(* Logix 5000 AddOnInstructionDefinition export NORD_ADC; software revision 24.02 *)

TYPE NORD_ParameterBackup :
STRUCT
   DeviceID : STRING;   // Device ID of VFD
   MacAddress : SINT[6];   // MAC Address of CU/TU
   ParamVFD : NORD_ParameterStoreInfo[1650];   // VFD Parameter Backup Values
   ParamCTU : NORD_ParameterStoreInfo[150];   // CU4/TU4 Parameter Backup Values
   HasIntPLC : BOOL;   // VFD contains an internal PLC Program
END_STRUCT
END_TYPE

TYPE NORD_ParameterStoreInfo :
STRUCT
   Num : INT;
   Inst : INT;
   Value : DINT;
END_STRUCT
END_TYPE

ADD_ON_INSTRUCTION NORD_ADC   (* revision 1.0, vendor NORD Drivesystems, ExecutePrescan, ExecuteEnableInFalse *)
// NORD ADC & Acyclic Comms.
// Revision note:
// For use with all NORD VFDs
//    - NORD Automatic Device Configurator
//       - Backup/Restore Parameters
//    - Acyclic Comms. for Parameter Read/Write
// Created By: Adam Desouky
VAR_IN_OUT
   ModuleName : MODULE; {required}
END_VAR
VAR_INPUT
   VFD_Number : SINT := 1; {visible}   // VFD Number in Localbus
   ParameterNumber : INT; {visible}
   ParameterIndex : SINT; {visible}
   ParameterSet : SINT; {visible}
END_VAR
VAR_OUTPUT
   Done : BOOL; {access Read Only, visible}
   Busy : BOOL; {access Read Only, visible}
END_VAR
VAR_IN_OUT
   ReadMsg : MESSAGE; {required}   // Read Msg to Module
END_VAR
VAR_INPUT
   ReadTrigger : BOOL; {visible}
   ReadValue : DINT; {access None, visible}   // Read Value from message
END_VAR
VAR_IN_OUT
   WriteMsg : MESSAGE; {required}   // Write Msg to Module
END_VAR
VAR_INPUT
   WriteTrigger : BOOL; {visible}
   WriteValue : DINT; {visible}
END_VAR
VAR_OUTPUT
   Error : BOOL; {access Read Only, visible}
   VFD_NotPresent : BOOL; {access Read Only, visible}   // VFD not present in Localbus
   EthernetDisconnected : BOOL; {access Read Only, visible}   // Eth. cord to Module is disconnected
END_VAR
VAR_IN_OUT
   Backup : NORD_ParameterBackup; {required}   // Parameter Backup File
END_VAR
VAR_OUTPUT
   CompletionPercent : DINT; {access None, visible}   // Backup/Restore Complete Percentage
   FirmwareUpdateRequired : BOOL; {access Read Only, visible}   // Parameter 780 not present
   NewDriveDetected : BOOL; {access Read Only, visible}   // New Device ID detected
   NewCTUnitDetected : BOOL; {access Read Only, visible}
END_VAR
VAR_INPUT
   BackupTrigger : BOOL; {visible}   // Trigger to start backing up the VFD parameters
   RestoreTrigger : BOOL; {visible}   // Trigger to start restoring the VFD parameters
   AutomaticRestore : BOOL; {access None, visible}   // Restore Automatically when New Drive is Detected
END_VAR
VAR_OUTPUT
   GetID_InProcess : BOOL; {access None, visible}
   BackupInProcess : BOOL; {access None, visible}
   RestoreInProcess : BOOL; {access None, visible}
   HasInternalPLC : BOOL; {access None, visible}
   ErrorID : DINT; {access Read Only, visible}   // Message Error Code
END_VAR
VAR_INPUT
   WriteValueMSG : DINT;
   ReadValueCarryOver : DINT; {access None}   // Do Not Delete
END_VAR
VAR
   ModulePath : SINT[32]; {access None}
   IP_Address : STRING; {access None}
   IP_Length : INT; {access None}
   Instance : INT;
   VFD_NumPrev : SINT := 1; {access None}
   VFD_NumLock : SINT := 1; {access None}
   GetID_SM : INT; {access None}   // 0: Not Active 10: Reset Info 20: Prepare Read Msg 30: Read Trigger 40: Read Complete 41: Store Data 42: Record Error 50: Increment Index 51: Switch to CU/TU
   HasParamIndex : BOOL; {access None}   // Set Parameter has Indexes
   HasParamSets : BOOL; {access None}   // Set Parameter has Parameter Sets
   ReadErrorOS : BOOL; {access None}
   WriteErrorONS : BOOL; {access None}
   TrigONS1 : BOOL; {access None}
   ReadDoneOS : BOOL; {access None}
   WriteDoneONS : BOOL; {access None}
   FaultCode : DINT; {access None}
   MacAddr : SINT[6]; {access None}   // MAC Address of CU/TU
   GetID_ReadTrigger : BOOL; {access None}
   EthConnONS : BOOL; {access None}
   GetID_DoneONS : BOOL; {access None}
   BackupSM : INT; {access None}   // 0: Not Active 10: Reset indexes 20: Clear Old Backup 30: Reset Indexes 40: Prepare Read Msg 50: Read Trigger 60: Read Complete 61: Store Data 70/71: Increment Store index/Instance 80: Increment Param 90: Store Device ID
   Index : INT; {access None}
   DeviceID : STRING; {access None}   // Device ID of VFD
   RestoreSM : INT; {access None}   // 0: Not Active 10: Reset Indexes 15: # of Saved Param 20: Get RestoreParam 21: Prepare Read Msg 22: Read Trigger 23: Read Complete 24: Compare Data 30: Prepare WriteMsg 40: Write Trigger 50: Write Complete 60: Inc. Store Index 70: Store Devide ID
   Index1 : INT; {access None}   // Store Index: VFD
   IndexInst : INT; {access None}   // Instance Index
   RestoreParam : INT := 5; {access None}   // Parameter Number to be Restored
   SavedParamsVFD : INT; {access None}
   MaxIndexVFD : INT; {access None}   // Maximun possible stored parameters
   BackupReadTrigger : BOOL; {access None}
   BackupIndexONS : BOOL; {access None}
   StartBackupONS : BOOL; {access None}
   RestWriteTrig : BOOL; {access None}
   RestIndexONS : BOOL; {access None}
   RestReadTrig : BOOL; {access None}
   BackupLast : BOOL; {access None}   // Determines Backup/Restore Complete Percentage Calculation
   WriteSM : SINT; {access None}   // 0: Not Active 10: Write LEN=4 20: 1st WriteTrigger 30: Write Complete - 40: Write LEN=2 - 50: 2nd WriteTrigger 60: Write Complete
   ID_Length : SINT := 12; {access None}
   Class : INT; {access None}
   TrigONS2 : BOOL; {access None}
   NullString : STRING; {access None}
   NumOfParams : DINT; {access None}   // Number of parameters in the VFD
   NewVFD_NumONS : BOOL; {access None}
   WriteTriggerONS : BOOL; {access None}
   WriteTrigInternal : BOOL; {access None}   // 1st Attempt: LEN = 4 2nd Attempt: LEN = 2
   Write16Bit : BOOL; {access None}   // 0: Write LEN=4 1: Write LEN=2
   AOI_FirstScan : BOOL; {access None}   // First Scan of AOI
   AOI_FirstScanONS : BOOL; {access None}
   Percent100ONS : BOOL; {access None}
   GetID_Done_ONS : BOOL; {access None}
   GetCTU_ID : BOOL; {access None}
   MaxIndexCTU : INT; {access None}
   Index2 : INT; {access None}   // Store Index: CU/TU
   SavedParamsCTU : INT; {access None}
   ID_Class : INT; {access None}
   RestoreCTU : BOOL; {access None}   // Restore CTU Parameters
   RestIndexONS2 : BOOL; {access None}
   ID_Attribute : INT; {access None}
   CompPercentIndex : INT; {access None}
   FirmwareONS : BOOL; {access None}
   StoreDevID : BOOL; {access None}
   StoreDevID_DN : BOOL; {access None}
   ResetIndexes : BOOL; {access None}
   ResetIndexDN : BOOL; {access None}
   GetRestParam : BOOL; {access None}   // Get Restore Parameter Logic
   GetRestParamDN : BOOL; {access None}   // Got Restore Param
   ClearDevID : BOOL; {access None}
   ClearDevID_DN : BOOL; {access None}
   ResetMsgEr : BOOL; {access None}
   ModuleEIP : BOOL; {access None}
   PerformRestoreONS : BOOL; {access None}
   RestoreFailed : BOOL; {access None}   // All writes in restore failed
   RestoreFailedONS : BOOL; {access None}
   RestoreHasWrite : BOOL; {access None}
   RestoreHasWriteONS : BOOL; {access None}
   AutomaticRestoreONS : BOOL; {access None}
   ModuleEIP_ONS : BOOL; {access None}
   GetID_Done : BOOL; {access None}
END_VAR

ROUTINE EnableInFalse   (* ladder *)
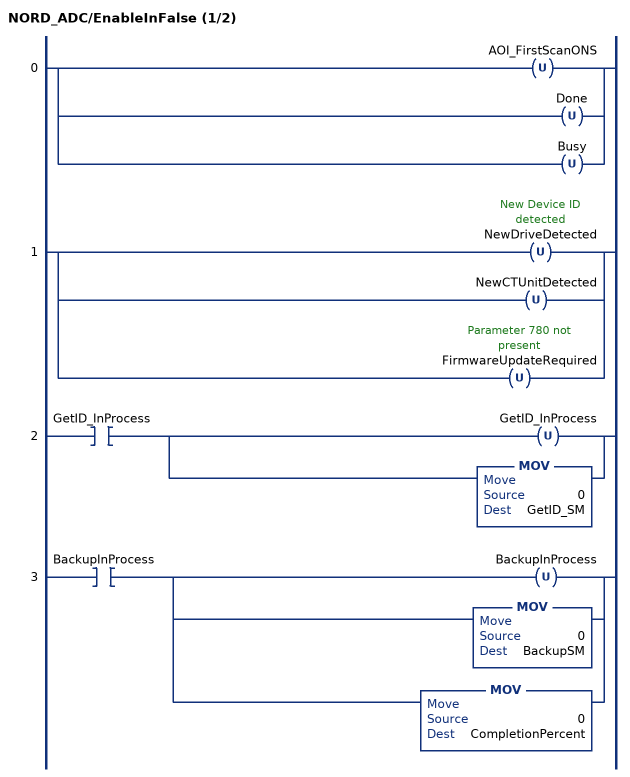
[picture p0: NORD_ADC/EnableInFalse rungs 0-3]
   0: [OTU(AOI_FirstScanONS) ,OTU(Done) ,OTU(Busy) ];
   1: [OTU(NewDriveDetected) ,OTU(NewCTUnitDetected) ,OTU(FirmwareUpdateRequired) ];
   2: XIC(GetID_InProcess)[OTU(GetID_InProcess) ,MOV(0,GetID_SM) ];
   3: XIC(BackupInProcess)[OTU(BackupInProcess) ,MOV(0,BackupSM) ,MOV(0,CompletionPercent) ];
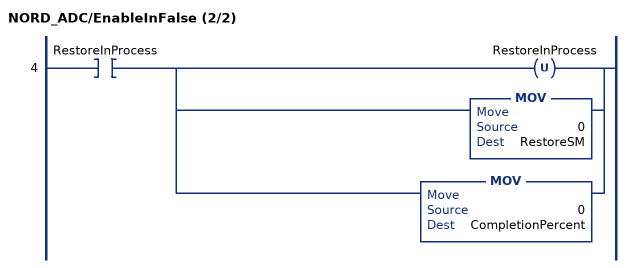
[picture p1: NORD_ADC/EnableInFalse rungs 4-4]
   4: XIC(RestoreInProcess)[OTU(RestoreInProcess) ,MOV(0,RestoreSM) ,MOV(0,CompletionPercent) ];
END_ROUTINE

ROUTINE Logic   (* ladder *)
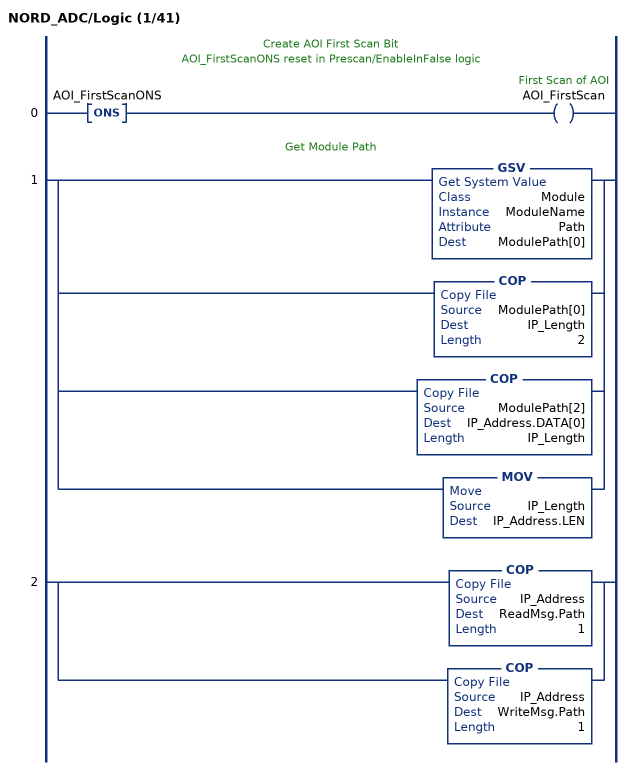
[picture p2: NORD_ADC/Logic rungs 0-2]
   // Create AOI First Scan Bit
   // AOI_FirstScanONS reset in Prescan/EnableInFalse logic
   0: ONS(AOI_FirstScanONS)OTE(AOI_FirstScan);
   // Get Module Path
   1: [GSV(Module,ModuleName,Path,ModulePath[0]) ,COP(ModulePath[0],IP_Length,2) ,COP(ModulePath[2],IP_Address.DATA[0],IP_Length) ,MOV(IP_Length,IP_Address.LEN) ];
   2: [COP(IP_Address,ReadMsg.Path,1) ,COP(IP_Address,WriteMsg.Path,1) ];
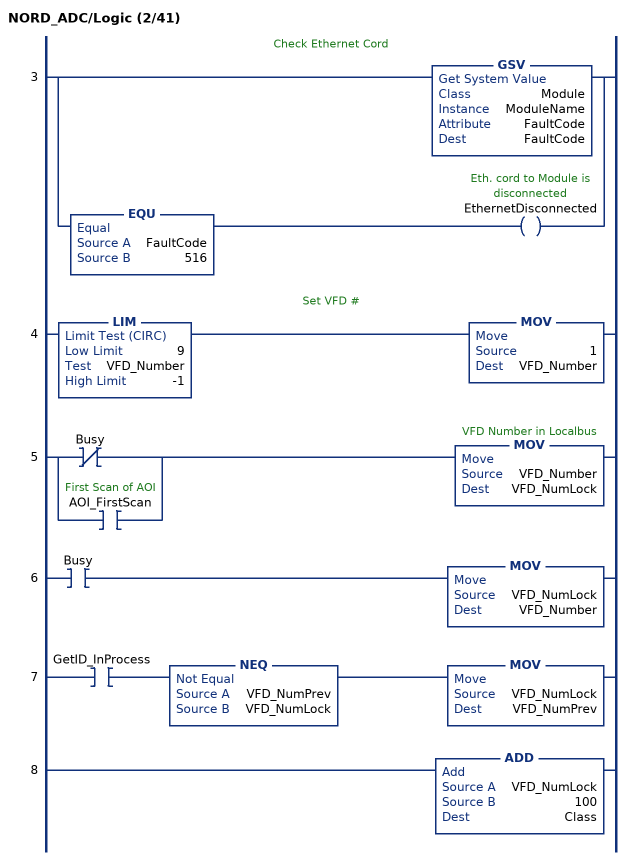
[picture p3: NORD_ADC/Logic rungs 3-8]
   // Check Ethernet Cord
   3: [GSV(Module,ModuleName,FaultCode,FaultCode) ,EQU(FaultCode,516) OTE(EthernetDisconnected) ];
   // Set VFD #
   4: LIM(9,VFD_Number,-1)MOV(1,VFD_Number);
   5: [XIO(Busy) ,XIC(AOI_FirstScan) ]MOV(VFD_Number,VFD_NumLock);
   6: XIC(Busy)MOV(VFD_NumLock,VFD_Number);
   7: XIC(GetID_InProcess)NEQ(VFD_NumPrev,VFD_NumLock)MOV(VFD_NumLock,VFD_NumPrev);
   8: ADD(VFD_NumLock,100,Class);
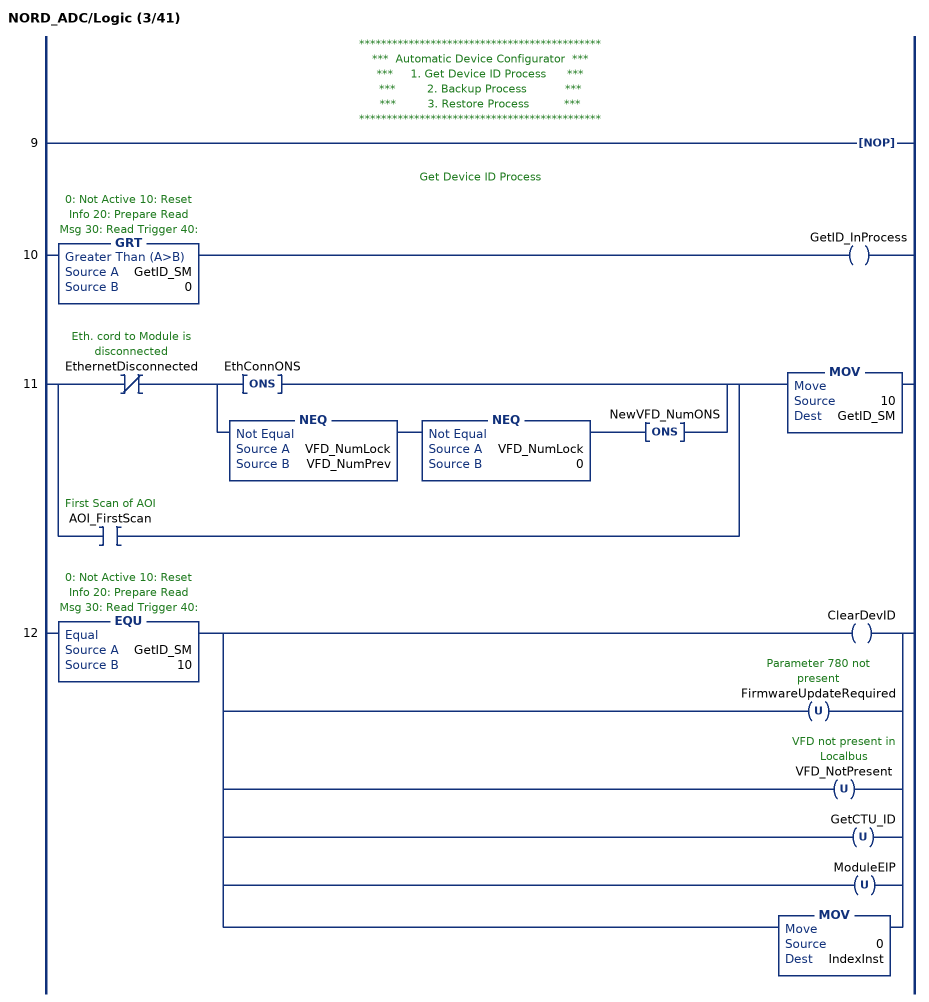
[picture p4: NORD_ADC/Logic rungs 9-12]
   // ********************************************
   // ***  Automatic Device Configurator  ***
   // ***     1. Get Device ID Process      ***
   // ***         2. Backup Process           ***
   // ***         3. Restore Process          ***
   // ********************************************
   9: NOP();
   // Get Device ID Process
   10: GRT(GetID_SM,0)OTE(GetID_InProcess);
   11: [XIO(EthernetDisconnected) [ONS(EthConnONS) ,NEQ(VFD_NumLock,VFD_NumPrev) NEQ(VFD_NumLock,0) ONS(NewVFD_NumONS) ] ,XIC(AOI_FirstScan) ]MOV(10,GetID_SM);
   12: EQU(GetID_SM,10)[OTE(ClearDevID) ,[OTU(FirmwareUpdateRequired) ,OTU(VFD_NotPresent) ,OTU(GetCTU_ID) ,OTU(ModuleEIP) ] ,MOV(0,IndexInst) ];
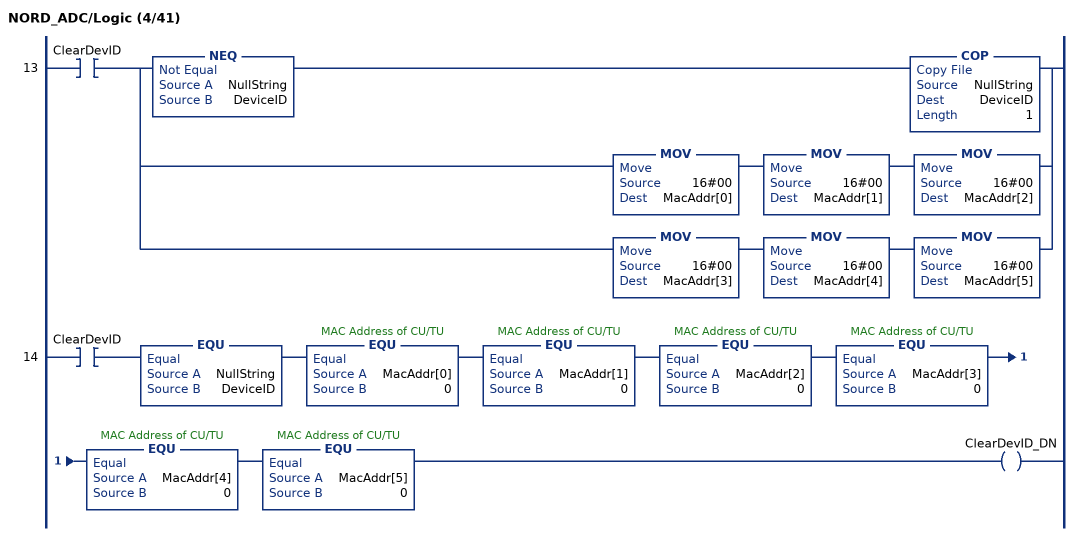
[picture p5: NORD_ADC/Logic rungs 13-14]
   13: XIC(ClearDevID)[NEQ(NullString,DeviceID) COP(NullString,DeviceID,1) ,MOV(16#00,MacAddr[0]) MOV(16#00,MacAddr[1]) MOV(16#00,MacAddr[2]) ,MOV(16#00,MacAddr[3]) MOV(16#00,MacAddr[4]) MOV(16#00,MacAddr[5]) ];
   14: XIC(ClearDevID)EQU(NullString,DeviceID)EQU(MacAddr[0],0)EQU(MacAddr[1],0)EQU(MacAddr[2],0)EQU(MacAddr[3],0)EQU(MacAddr[4],0)EQU(MacAddr[5],0)OTE(ClearDevID_DN);
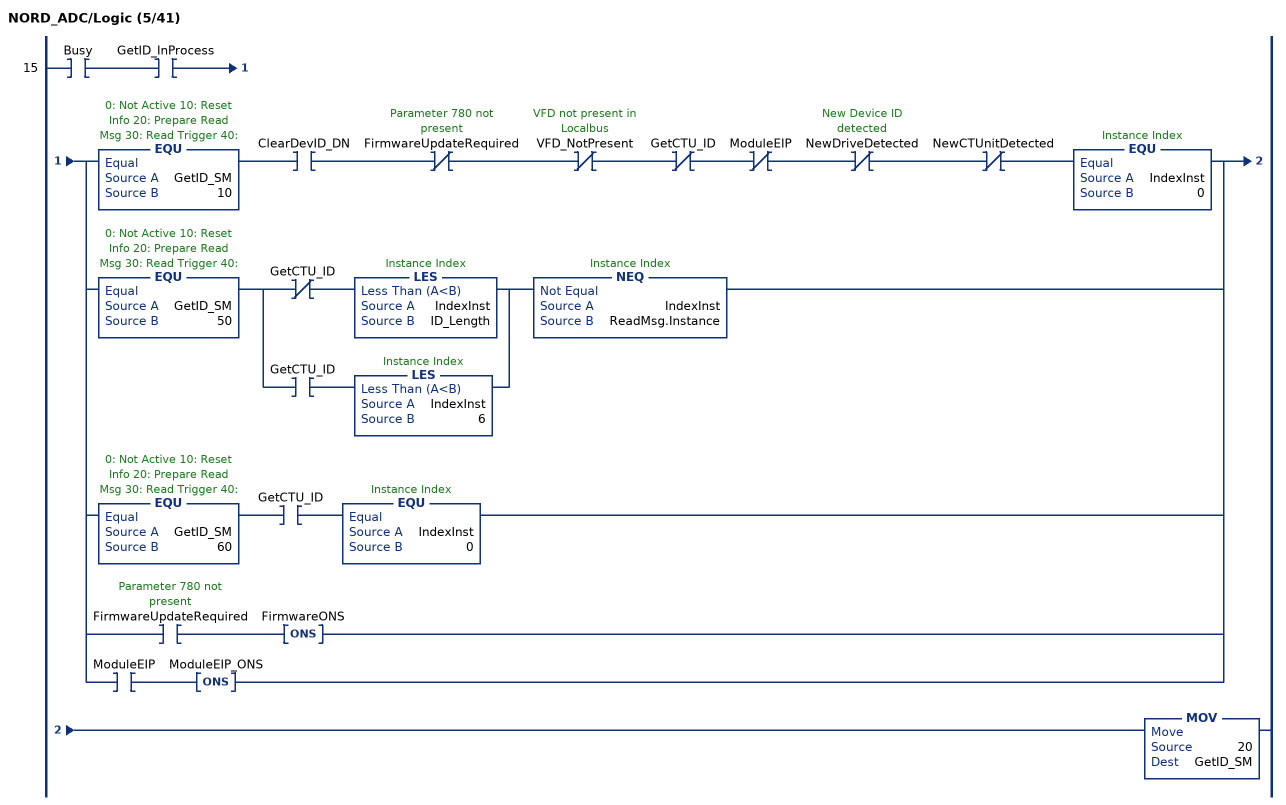
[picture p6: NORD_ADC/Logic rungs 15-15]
   15: XIC(Busy)XIC(GetID_InProcess)[EQU(GetID_SM,10) XIC(ClearDevID_DN) XIO(FirmwareUpdateRequired) XIO(VFD_NotPresent) XIO(GetCTU_ID) XIO(ModuleEIP) XIO(NewDriveDetected) XIO(NewCTUnitDetected) EQU(IndexInst,0) ,EQU(GetID_SM,50) [XIO(GetCTU_ID) LES(IndexInst,ID_Length) ,XIC(GetCTU_ID) LES(IndexInst,6) ] NEQ(IndexInst,ReadMsg.Instance) ,EQU(GetID_SM,60) XIC(GetCTU_ID) EQU(IndexInst,0) ,XIC(FirmwareUpdateRequired) ONS(FirmwareONS) ,XIC(ModuleEIP) ONS(ModuleEIP_ONS) ]MOV(20,GetID_SM);
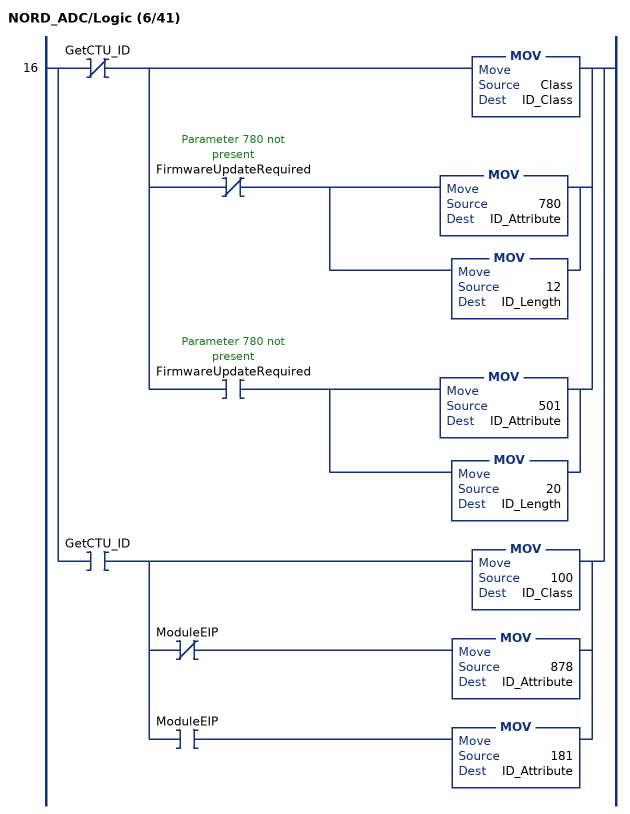
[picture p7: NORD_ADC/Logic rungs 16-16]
   16: [XIO(GetCTU_ID) [MOV(Class,ID_Class) ,XIO(FirmwareUpdateRequired) [MOV(780,ID_Attribute) ,MOV(12,ID_Length) ] ,XIC(FirmwareUpdateRequired) [MOV(501,ID_Attribute) ,MOV(20,ID_Length) ] ] ,XIC(GetCTU_ID) [MOV(100,ID_Class) ,XIO(ModuleEIP) MOV(878,ID_Attribute) ,XIC(ModuleEIP) MOV(181,ID_Attribute) ] ];
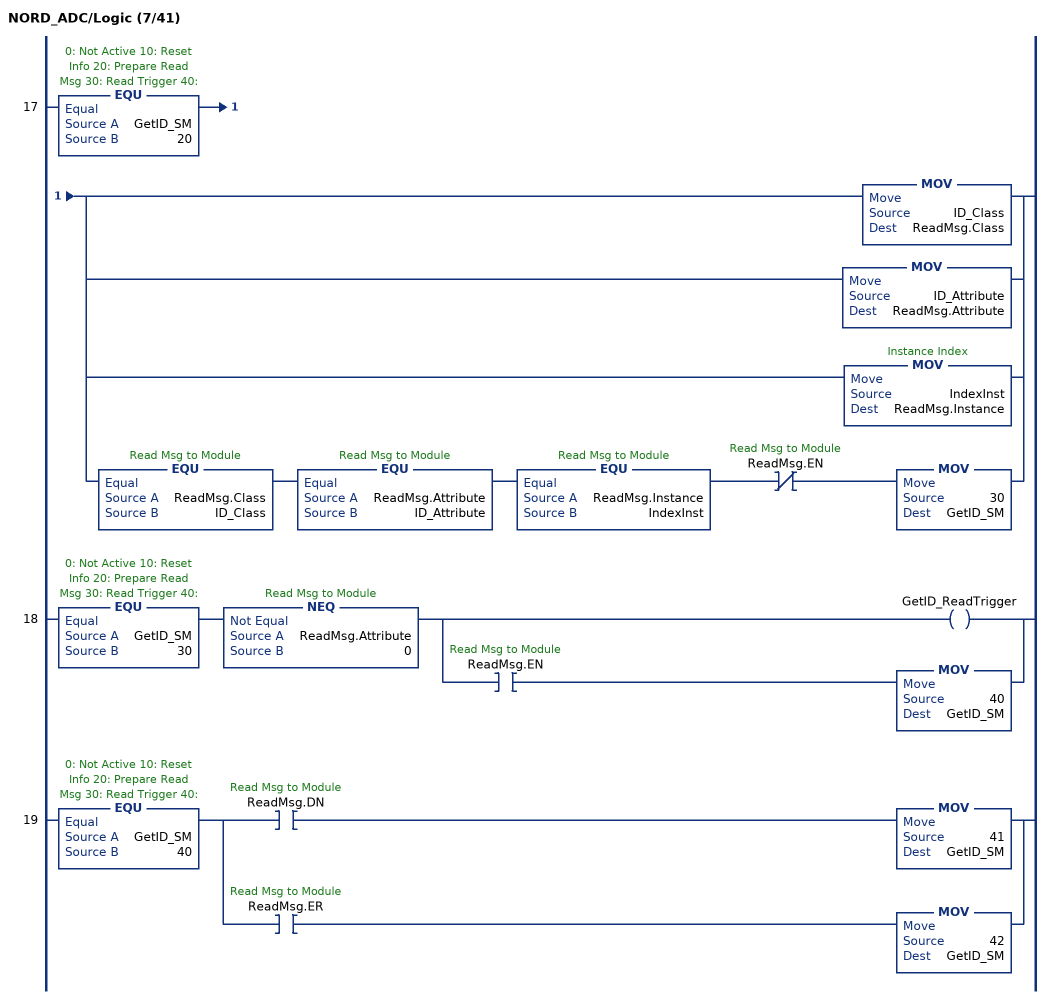
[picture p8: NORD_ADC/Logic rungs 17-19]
   17: EQU(GetID_SM,20)[[MOV(ID_Class,ReadMsg.Class) ,MOV(ID_Attribute,ReadMsg.Attribute) ,MOV(IndexInst,ReadMsg.Instance) ] ,EQU(ReadMsg.Class,ID_Class) EQU(ReadMsg.Attribute,ID_Attribute) EQU(ReadMsg.Instance,IndexInst) XIO(ReadMsg.EN) MOV(30,GetID_SM) ];
   18: EQU(GetID_SM,30)NEQ(ReadMsg.Attribute,0)[OTE(GetID_ReadTrigger) ,XIC(ReadMsg.EN) MOV(40,GetID_SM) ];
   19: EQU(GetID_SM,40)[XIC(ReadMsg.DN) MOV(41,GetID_SM) ,XIC(ReadMsg.ER) MOV(42,GetID_SM) ];
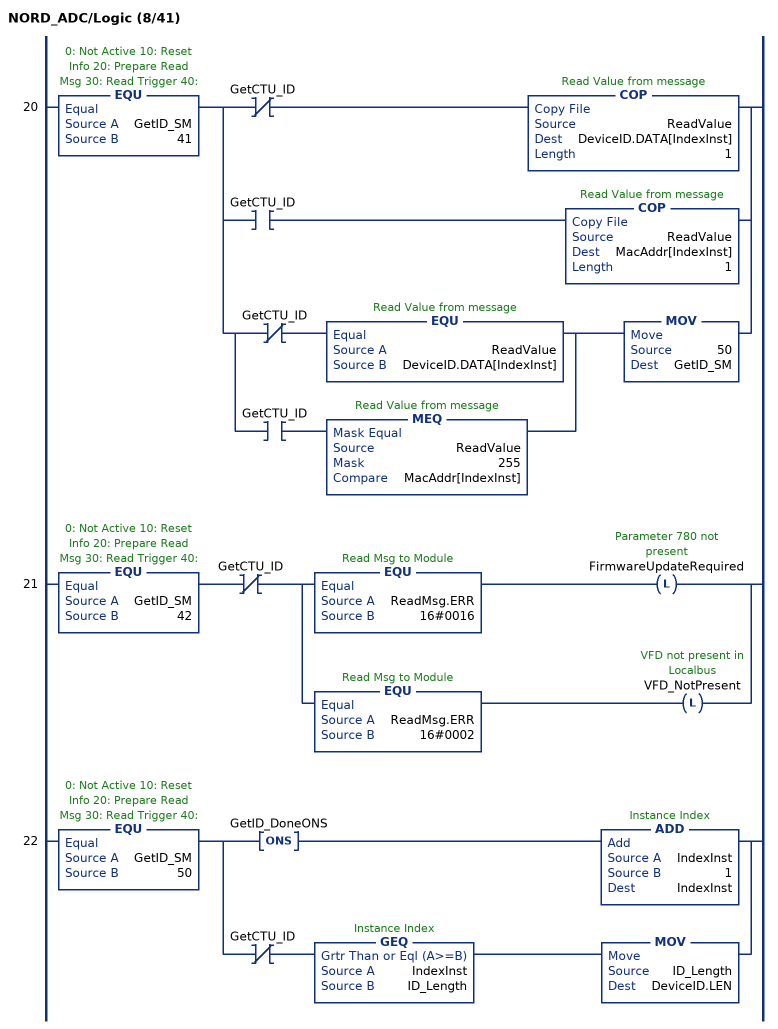
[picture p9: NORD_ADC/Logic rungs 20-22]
   20: EQU(GetID_SM,41)[[XIO(GetCTU_ID) COP(ReadValue,DeviceID.DATA[IndexInst],1) ,XIC(GetCTU_ID) COP(ReadValue,MacAddr[IndexInst],1) ] ,[XIO(GetCTU_ID) EQU(ReadValue,DeviceID.DATA[IndexInst]) ,XIC(GetCTU_ID) MEQ(ReadValue,255,MacAddr[IndexInst]) ] MOV(50,GetID_SM) ];
   21: EQU(GetID_SM,42)XIO(GetCTU_ID)[EQU(ReadMsg.ERR,16#0016) OTL(FirmwareUpdateRequired) ,EQU(ReadMsg.ERR,16#0002) OTL(VFD_NotPresent) ];
   22: EQU(GetID_SM,50)[ONS(GetID_DoneONS) ADD(IndexInst,1,IndexInst) ,XIO(GetCTU_ID) GEQ(IndexInst,ID_Length) MOV(ID_Length,DeviceID.LEN) ];
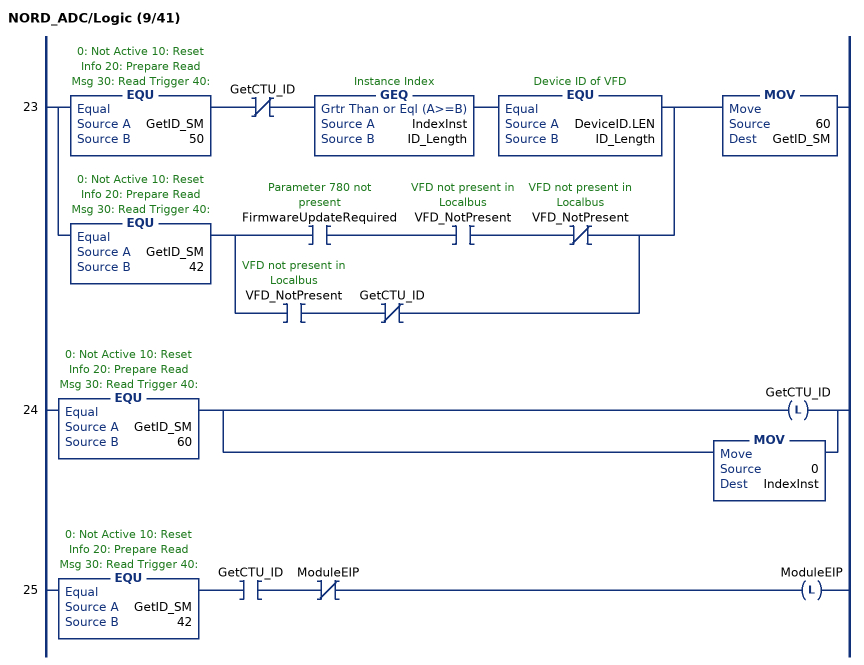
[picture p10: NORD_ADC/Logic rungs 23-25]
   23: [EQU(GetID_SM,50) XIO(GetCTU_ID) GEQ(IndexInst,ID_Length) EQU(DeviceID.LEN,ID_Length) ,EQU(GetID_SM,42) [XIC(FirmwareUpdateRequired) XIC(VFD_NotPresent) XIO(VFD_NotPresent) ,XIC(VFD_NotPresent) XIO(GetCTU_ID) ] ]MOV(60,GetID_SM);
   24: EQU(GetID_SM,60)[OTL(GetCTU_ID) ,MOV(0,IndexInst) ];
   25: EQU(GetID_SM,42)XIC(GetCTU_ID)XIO(ModuleEIP)OTL(ModuleEIP);
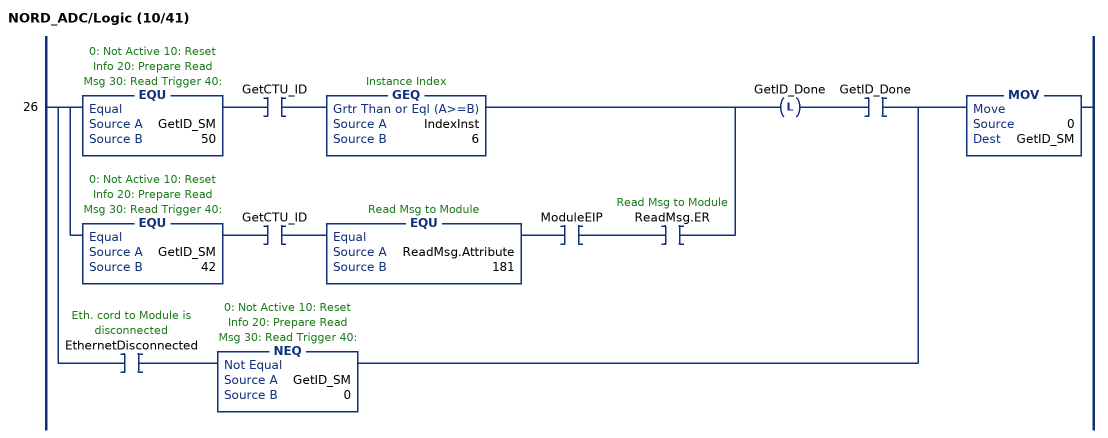
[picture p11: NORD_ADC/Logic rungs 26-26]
   26: [[EQU(GetID_SM,50) XIC(GetCTU_ID) GEQ(IndexInst,6) ,EQU(GetID_SM,42) XIC(GetCTU_ID) EQU(ReadMsg.Attribute,181) XIC(ModuleEIP) XIC(ReadMsg.ER) ] OTL(GetID_Done) XIC(GetID_Done) ,XIC(EthernetDisconnected) NEQ(GetID_SM,0) ]MOV(0,GetID_SM);
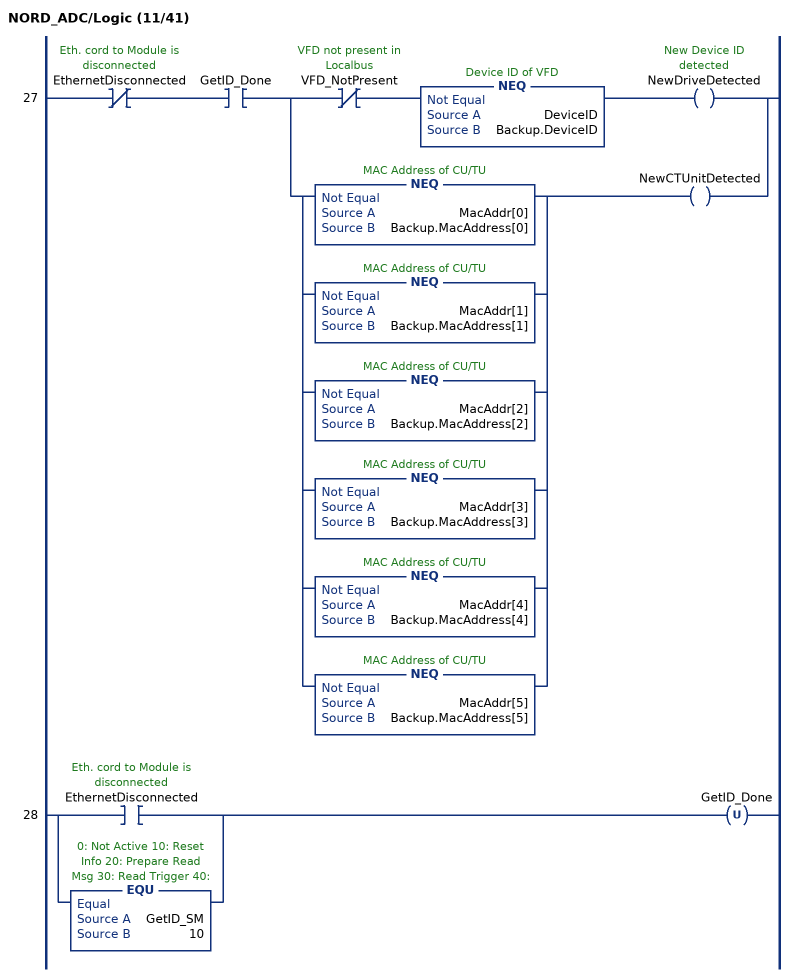
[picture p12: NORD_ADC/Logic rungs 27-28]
   27: XIO(EthernetDisconnected)XIC(GetID_Done)[XIO(VFD_NotPresent) NEQ(DeviceID,Backup.DeviceID) OTE(NewDriveDetected) ,[NEQ(MacAddr[0],Backup.MacAddress[0]) ,NEQ(MacAddr[1],Backup.MacAddress[1]) ,NEQ(MacAddr[2],Backup.MacAddress[2]) ,NEQ(MacAddr[3],Backup.MacAddress[3]) ,NEQ(MacAddr[4],Backup.MacAddress[4]) ,NEQ(MacAddr[5],Backup.MacAddress[5]) ] OTE(NewCTUnitDetected) ];
   28: [XIC(EthernetDisconnected) ,EQU(GetID_SM,10) ]OTU(GetID_Done);
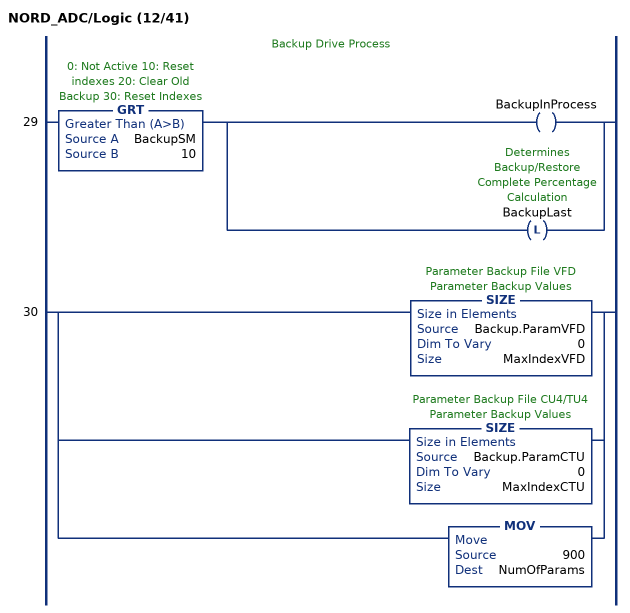
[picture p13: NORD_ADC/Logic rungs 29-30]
   // Backup Drive Process
   29: GRT(BackupSM,10)[OTE(BackupInProcess) ,OTL(BackupLast) ];
   30: [SIZE(Backup.ParamVFD,0,MaxIndexVFD) ,SIZE(Backup.ParamCTU,0,MaxIndexCTU) ,MOV(900,NumOfParams) ];
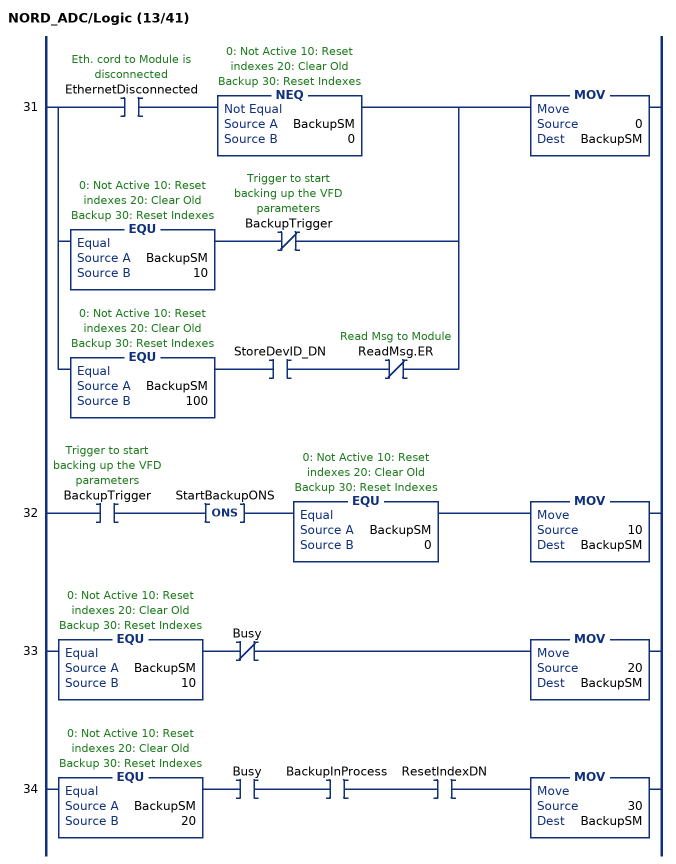
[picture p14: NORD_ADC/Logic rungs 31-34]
   31: [XIC(EthernetDisconnected) NEQ(BackupSM,0) ,EQU(BackupSM,10) XIO(BackupTrigger) ,EQU(BackupSM,100) XIC(StoreDevID_DN) XIO(ReadMsg.ER) ]MOV(0,BackupSM);
   32: XIC(BackupTrigger)ONS(StartBackupONS)EQU(BackupSM,0)MOV(10,BackupSM);
   33: EQU(BackupSM,10)XIO(Busy)MOV(20,BackupSM);
   34: EQU(BackupSM,20)XIC(Busy)XIC(BackupInProcess)XIC(ResetIndexDN)MOV(30,BackupSM);
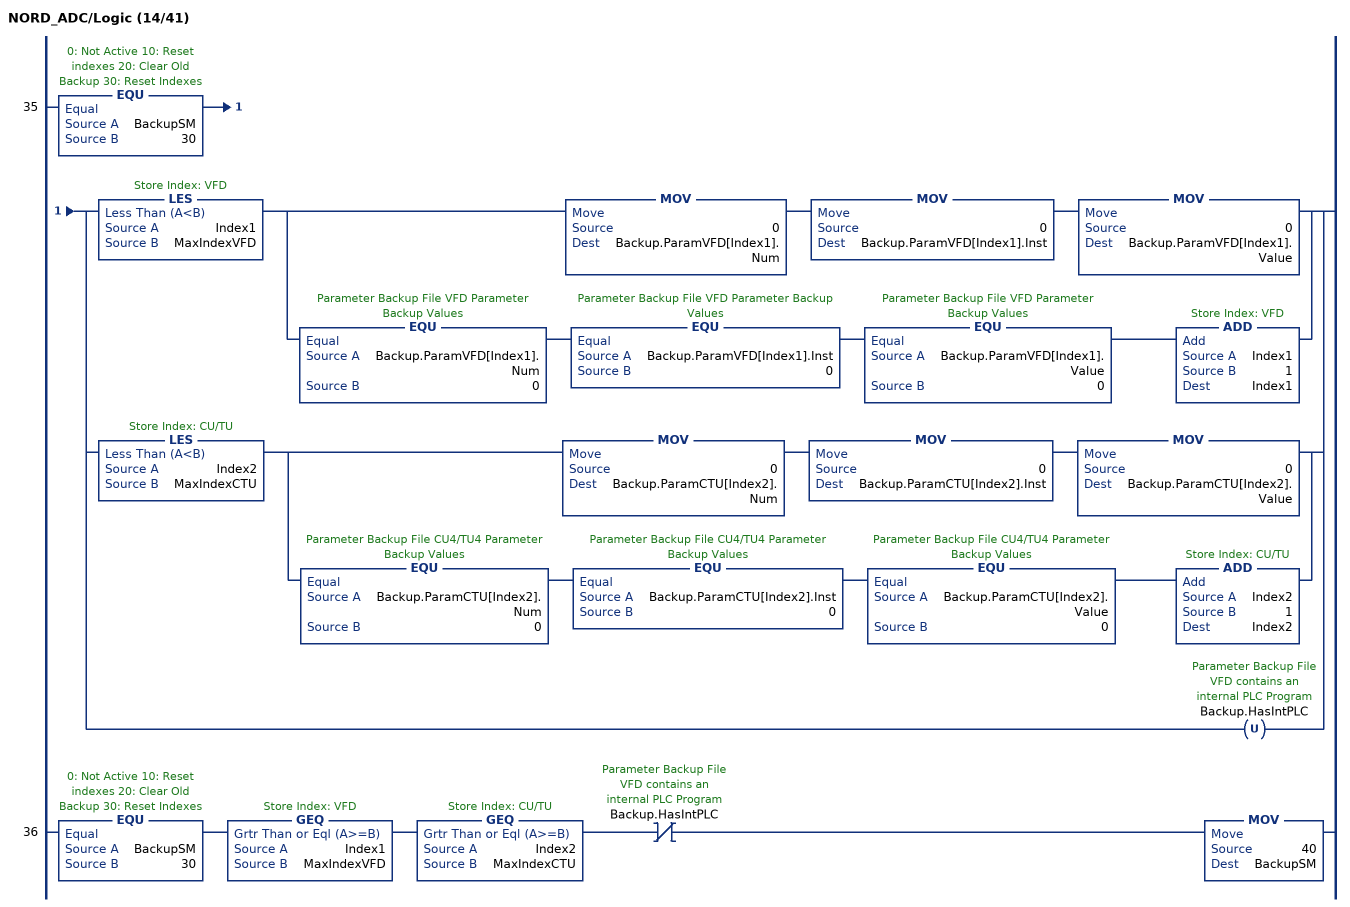
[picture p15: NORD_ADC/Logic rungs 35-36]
   35: EQU(BackupSM,30)[LES(Index1,MaxIndexVFD) [MOV(0,Backup.ParamVFD[Index1].Num) MOV(0,Backup.ParamVFD[Index1].Inst) MOV(0,Backup.ParamVFD[Index1].Value) ,EQU(Backup.ParamVFD[Index1].Num,0) EQU(Backup.ParamVFD[Index1].Inst,0) EQU(Backup.ParamVFD[Index1].Value,0) ADD(Index1,1,Index1) ] ,LES(Index2,MaxIndexCTU) [MOV(0,Backup.ParamCTU[Index2].Num) MOV(0,Backup.ParamCTU[Index2].Inst) MOV(0,Backup.ParamCTU[Index2].Value) ,EQU(Backup.ParamCTU[Index2].Num,0) EQU(Backup.ParamCTU[Index2].Inst,0) EQU(Backup.ParamCTU[Index2].Value,0) ADD(Index2,1,Index2) ] ,OTU(Backup.HasIntPLC) ];
   36: EQU(BackupSM,30)GEQ(Index1,MaxIndexVFD)GEQ(Index2,MaxIndexCTU)XIO(Backup.HasIntPLC)MOV(40,BackupSM);
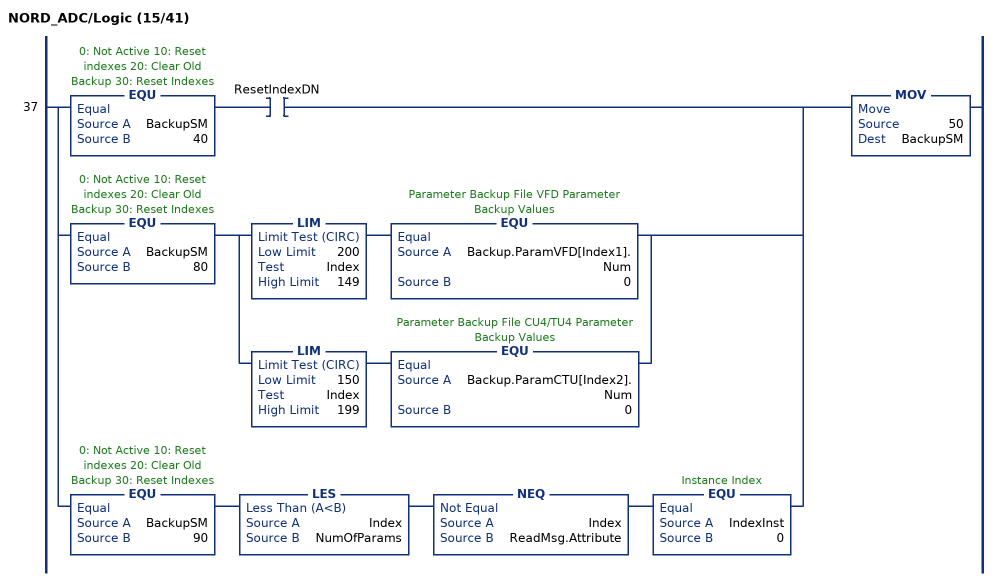
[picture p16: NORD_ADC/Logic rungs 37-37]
   37: [EQU(BackupSM,40) XIC(ResetIndexDN) ,EQU(BackupSM,80) [LIM(200,Index,149) EQU(Backup.ParamVFD[Index1].Num,0) ,LIM(150,Index,199) EQU(Backup.ParamCTU[Index2].Num,0) ] ,EQU(BackupSM,90) LES(Index,NumOfParams) NEQ(Index,ReadMsg.Attribute) EQU(IndexInst,0) ]MOV(50,BackupSM);
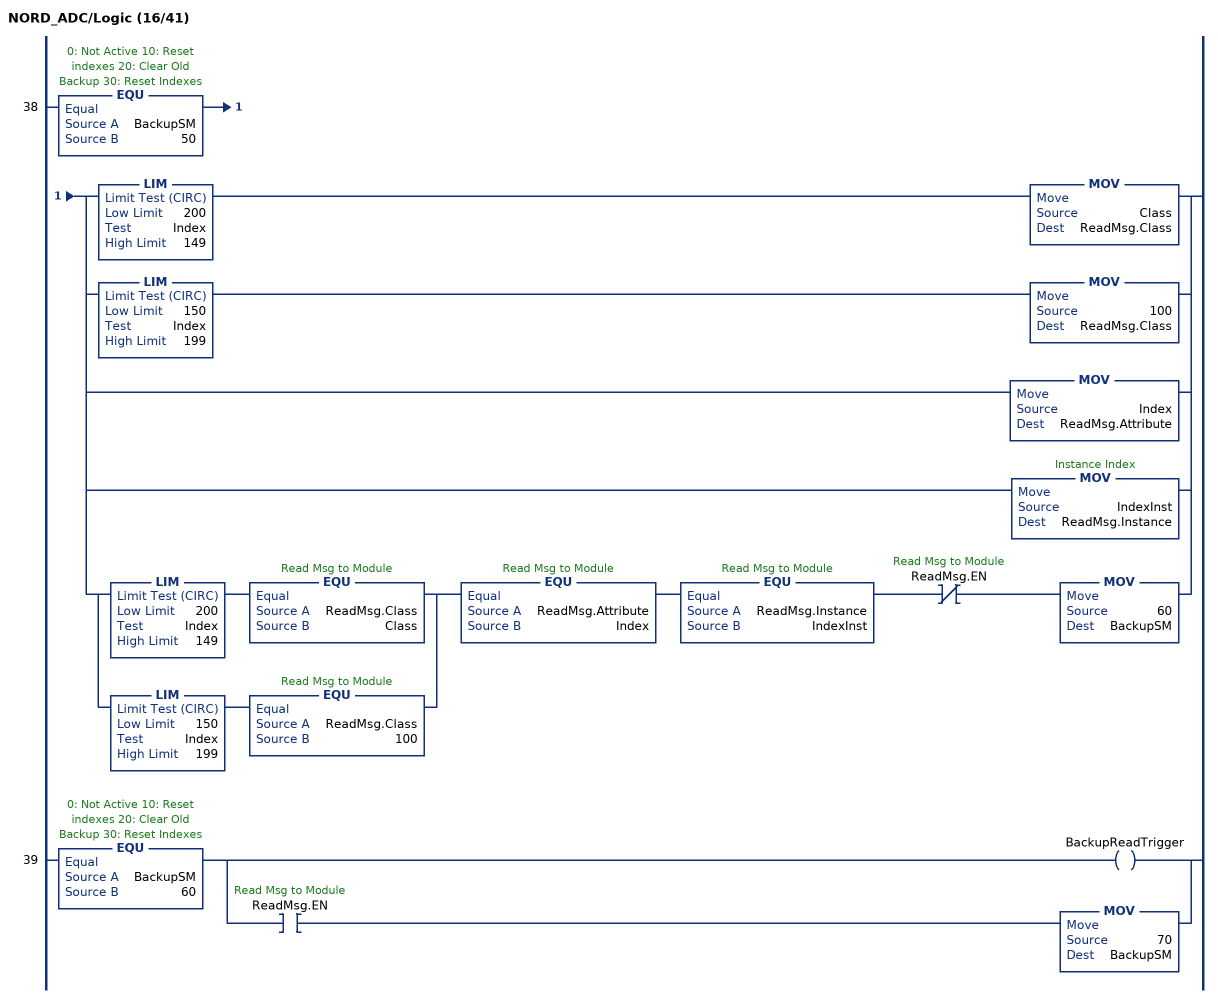
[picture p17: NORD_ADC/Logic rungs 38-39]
   38: EQU(BackupSM,50)[[LIM(200,Index,149) MOV(Class,ReadMsg.Class) ,LIM(150,Index,199) MOV(100,ReadMsg.Class) ] ,MOV(Index,ReadMsg.Attribute) ,MOV(IndexInst,ReadMsg.Instance) ,[LIM(200,Index,149) EQU(ReadMsg.Class,Class) ,LIM(150,Index,199) EQU(ReadMsg.Class,100) ] EQU(ReadMsg.Attribute,Index) EQU(ReadMsg.Instance,IndexInst) XIO(ReadMsg.EN) MOV(60,BackupSM) ];
   39: EQU(BackupSM,60)[OTE(BackupReadTrigger) ,XIC(ReadMsg.EN) MOV(70,BackupSM) ];
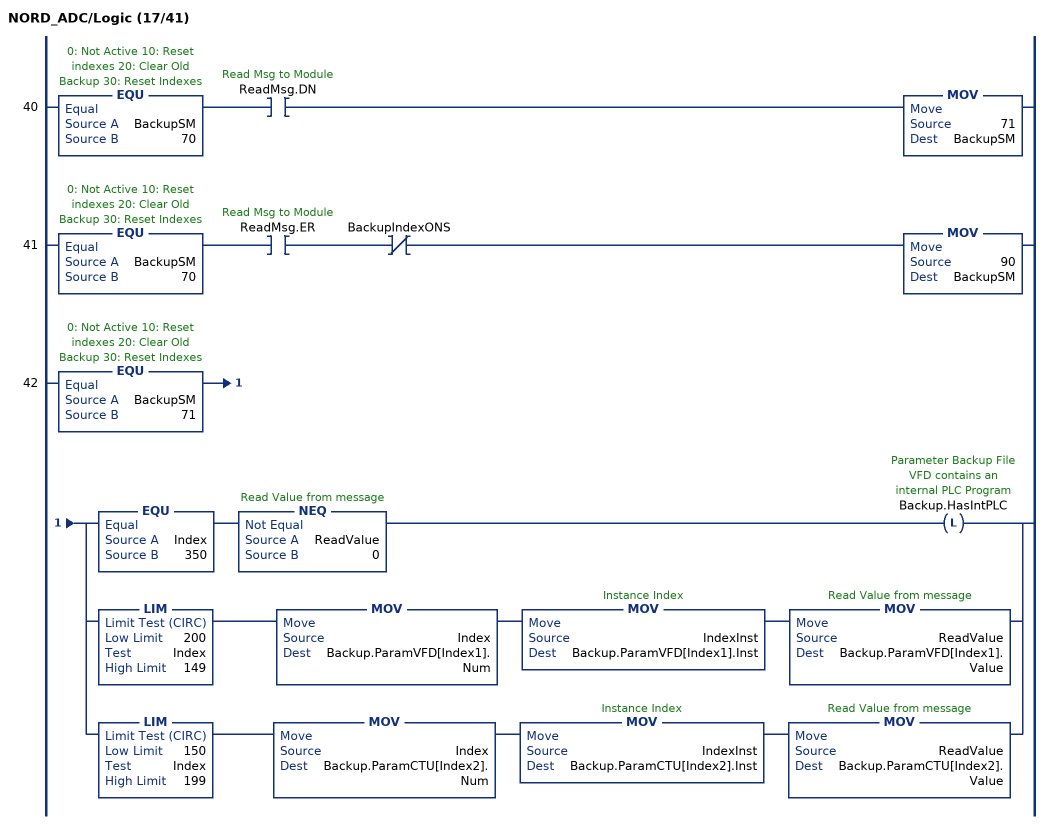
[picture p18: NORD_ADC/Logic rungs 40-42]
   40: EQU(BackupSM,70)XIC(ReadMsg.DN)MOV(71,BackupSM);
   41: EQU(BackupSM,70)XIC(ReadMsg.ER)XIO(BackupIndexONS)MOV(90,BackupSM);
   42: EQU(BackupSM,71)[EQU(Index,350) NEQ(ReadValue,0) OTL(Backup.HasIntPLC) ,LIM(200,Index,149) MOV(Index,Backup.ParamVFD[Index1].Num) MOV(IndexInst,Backup.ParamVFD[Index1].Inst) MOV(ReadValue,Backup.ParamVFD[Index1].Value) ,LIM(150,Index,199) MOV(Index,Backup.ParamCTU[Index2].Num) MOV(IndexInst,Backup.ParamCTU[Index2].Inst) MOV(ReadValue,Backup.ParamCTU[Index2].Value) ];
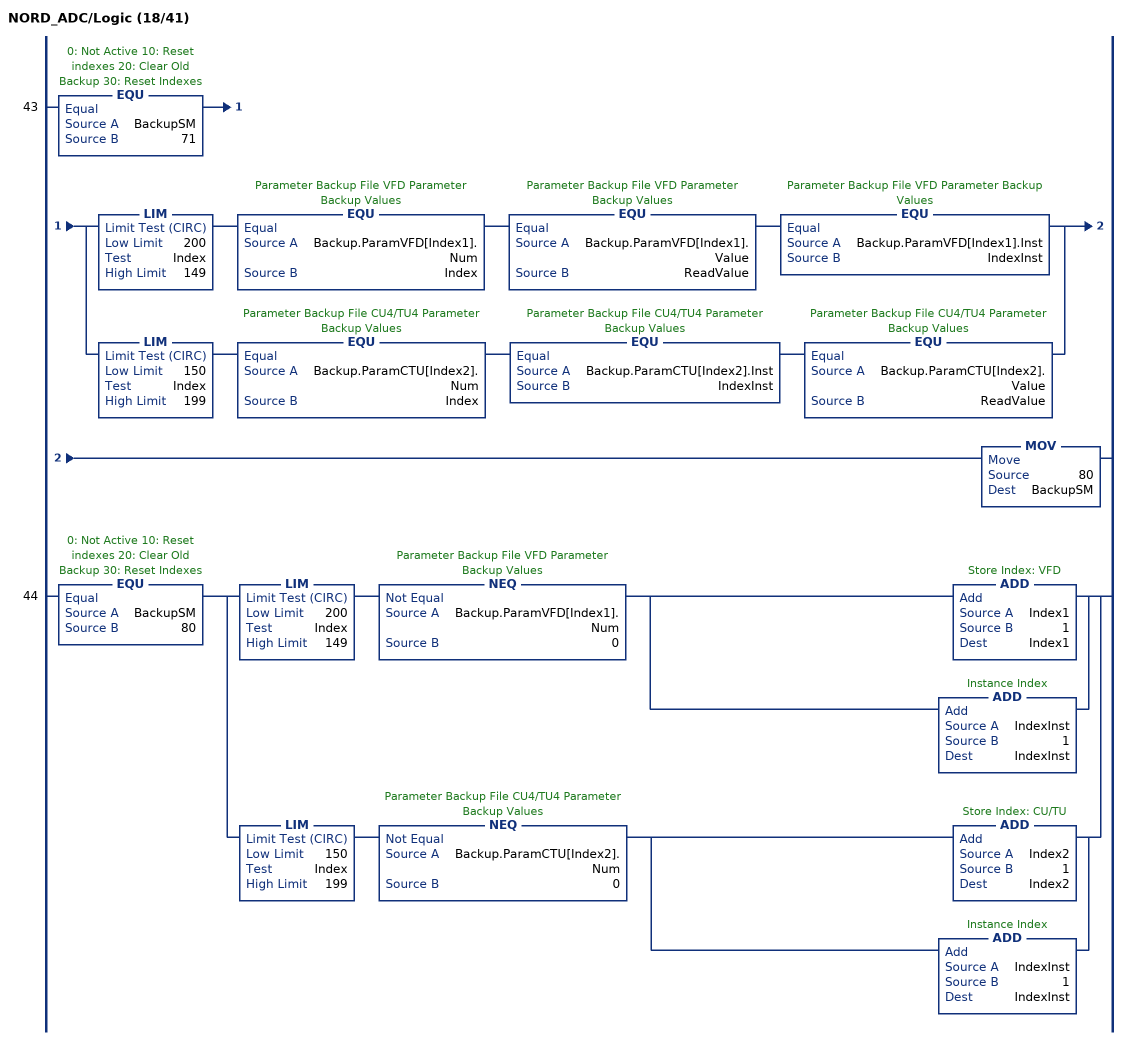
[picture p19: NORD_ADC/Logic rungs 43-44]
   43: EQU(BackupSM,71)[LIM(200,Index,149) EQU(Backup.ParamVFD[Index1].Num,Index) EQU(Backup.ParamVFD[Index1].Value,ReadValue) EQU(Backup.ParamVFD[Index1].Inst,IndexInst) ,LIM(150,Index,199) EQU(Backup.ParamCTU[Index2].Num,Index) EQU(Backup.ParamCTU[Index2].Inst,IndexInst) EQU(Backup.ParamCTU[Index2].Value,ReadValue) ]MOV(80,BackupSM);
   44: EQU(BackupSM,80)[LIM(200,Index,149) NEQ(Backup.ParamVFD[Index1].Num,0) [ADD(Index1,1,Index1) ,ADD(IndexInst,1,IndexInst) ] ,LIM(150,Index,199) NEQ(Backup.ParamCTU[Index2].Num,0) [ADD(Index2,1,Index2) ,ADD(IndexInst,1,IndexInst) ] ];
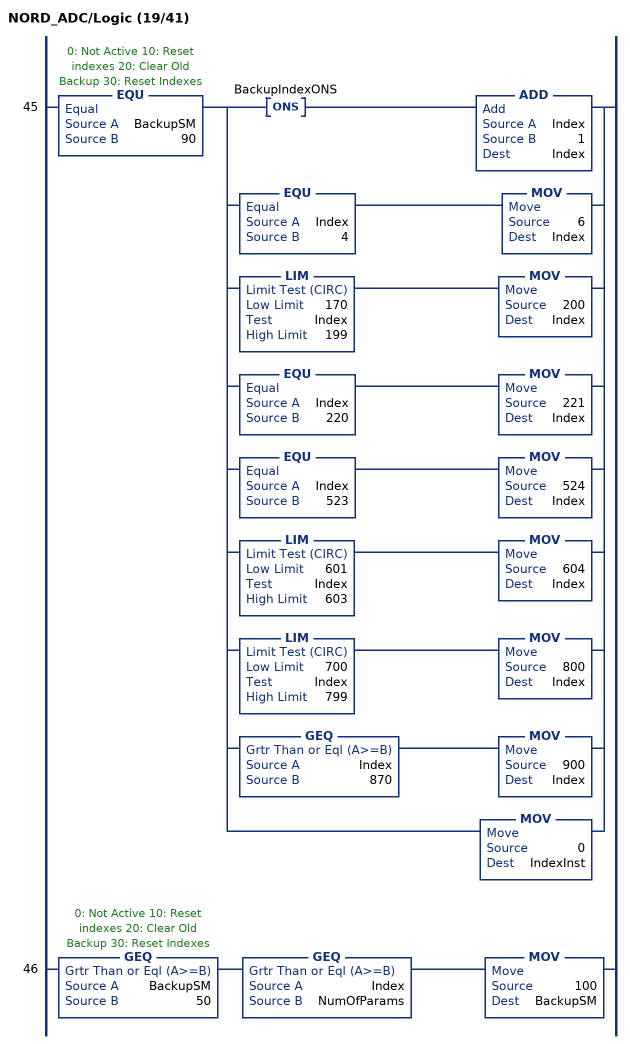
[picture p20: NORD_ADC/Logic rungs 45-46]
   45: EQU(BackupSM,90)[ONS(BackupIndexONS) ADD(Index,1,Index) ,EQU(Index,4) MOV(6,Index) ,LIM(170,Index,199) MOV(200,Index) ,EQU(Index,220) MOV(221,Index) ,EQU(Index,523) MOV(524,Index) ,LIM(601,Index,603) MOV(604,Index) ,LIM(700,Index,799) MOV(800,Index) ,GEQ(Index,870) MOV(900,Index) ,MOV(0,IndexInst) ];
   46: GEQ(BackupSM,50)GEQ(Index,NumOfParams)MOV(100,BackupSM);
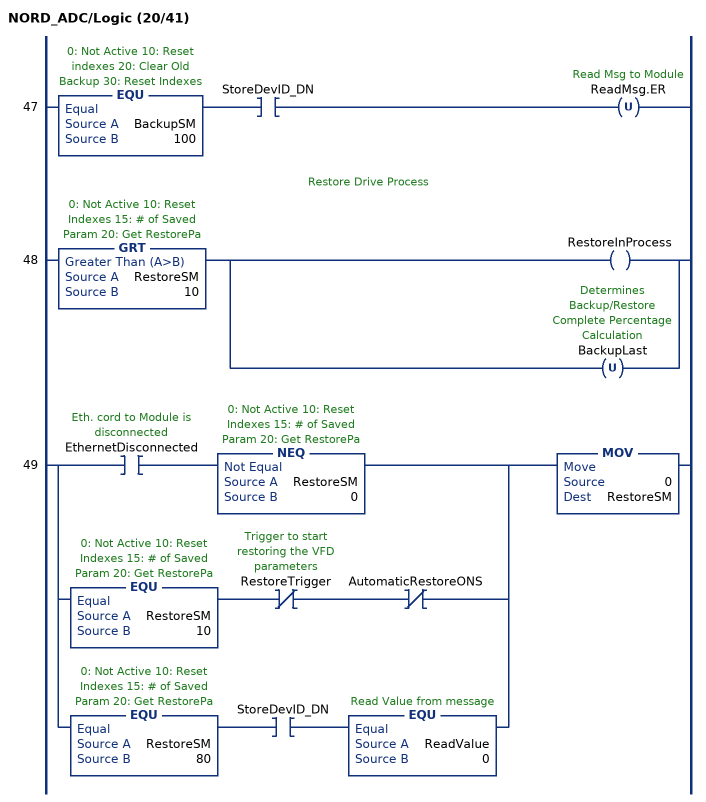
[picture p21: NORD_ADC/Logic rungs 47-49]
   47: EQU(BackupSM,100)XIC(StoreDevID_DN)OTU(ReadMsg.ER);
   // Restore Drive Process
   48: GRT(RestoreSM,10)[OTE(RestoreInProcess) ,OTU(BackupLast) ];
   49: [XIC(EthernetDisconnected) NEQ(RestoreSM,0) ,EQU(RestoreSM,10) XIO(RestoreTrigger) XIO(AutomaticRestoreONS) ,EQU(RestoreSM,80) XIC(StoreDevID_DN) EQU(ReadValue,0) ]MOV(0,RestoreSM);
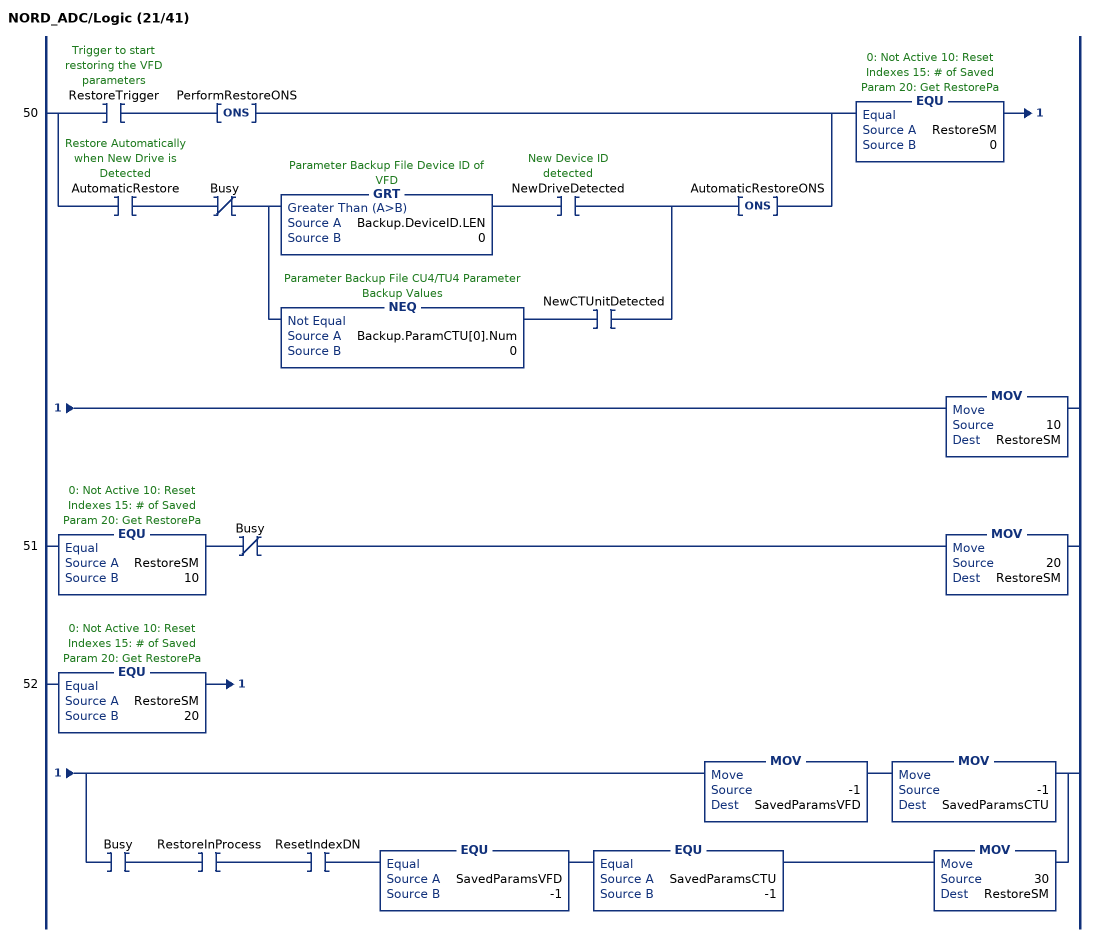
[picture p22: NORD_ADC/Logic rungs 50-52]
   50: [XIC(RestoreTrigger) ONS(PerformRestoreONS) ,XIC(AutomaticRestore) XIO(Busy) [GRT(Backup.DeviceID.LEN,0) XIC(NewDriveDetected) ,NEQ(Backup.ParamCTU[0].Num,0) XIC(NewCTUnitDetected) ] ONS(AutomaticRestoreONS) ]EQU(RestoreSM,0)MOV(10,RestoreSM);
   51: EQU(RestoreSM,10)XIO(Busy)MOV(20,RestoreSM);
   52: EQU(RestoreSM,20)[MOV(-1,SavedParamsVFD) MOV(-1,SavedParamsCTU) ,XIC(Busy) XIC(RestoreInProcess) XIC(ResetIndexDN) EQU(SavedParamsVFD,-1) EQU(SavedParamsCTU,-1) MOV(30,RestoreSM) ];
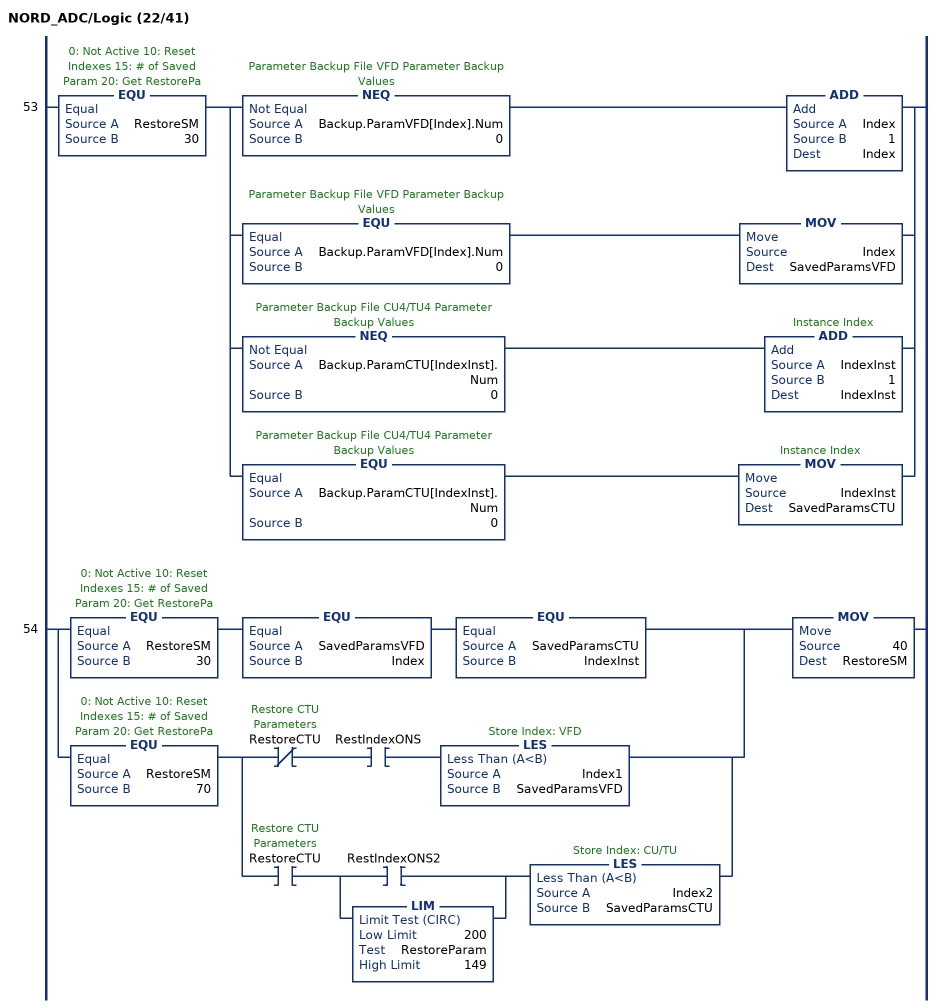
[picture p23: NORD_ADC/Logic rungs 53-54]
   53: EQU(RestoreSM,30)[[NEQ(Backup.ParamVFD[Index].Num,0) ADD(Index,1,Index) ,EQU(Backup.ParamVFD[Index].Num,0) MOV(Index,SavedParamsVFD) ] ,[NEQ(Backup.ParamCTU[IndexInst].Num,0) ADD(IndexInst,1,IndexInst) ,EQU(Backup.ParamCTU[IndexInst].Num,0) MOV(IndexInst,SavedParamsCTU) ] ];
   54: [EQU(RestoreSM,30) EQU(SavedParamsVFD,Index) EQU(SavedParamsCTU,IndexInst) ,EQU(RestoreSM,70) [XIO(RestoreCTU) XIC(RestIndexONS) LES(Index1,SavedParamsVFD) ,XIC(RestoreCTU) [XIC(RestIndexONS2) ,LIM(200,RestoreParam,149) ] LES(Index2,SavedParamsCTU) ] ]MOV(40,RestoreSM);
